TYPE ST_ChildStructure :
STRUCT
	{attribute 'ElementName' := 'Name'}
    Name : STRING(256);
	{attribute 'ElementName' := 'Value'}
	Value: LINT;
	{attribute 'ElementName' := 'myBool'}
	myBool : BOOL;
	{attribute 'ElementName' := 'arr'}
	arr : ARRAY[0..3] OF LREAL;
	{attribute 'ElementName' := 'myBool2'}
	myBool2 : BOOL; 
END_STRUCT
END_TYPE
